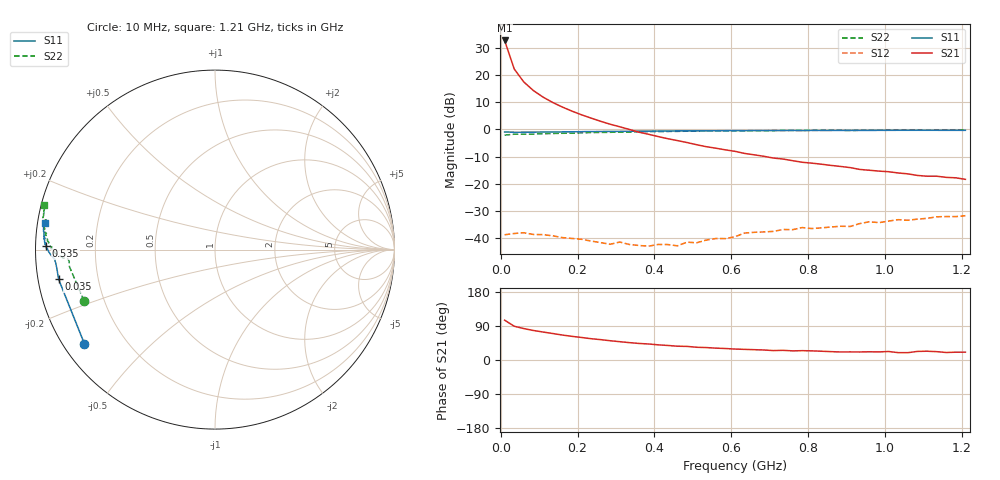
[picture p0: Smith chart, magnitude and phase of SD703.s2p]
!  POLYFET RF DEVICES
!  S PARAMETERS FOR
!  SD703 (EACH SIDE)
!  VDS=28, IDQ=600MA
! S1A3Die Vds=28Vdc, Idq=600ma, Vgsth=2.63Vdc
! Date: Thu Jul 23 11:57:09 1998
# MHZ  S  MA  R  50.0000
! SCATTERING PARAMETERS :
! Freq=MHz Mag[s11] Ang[s11] Mag[s21] Ang[s21] Mag[s12] Ang[s12] Mag[s22] Ang[s22]
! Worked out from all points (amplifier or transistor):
!   49 points, 10 MHz to 1.21 GHz, reference 50 ohm
!   highest |S21| = 32.7 dB at 10 MHz (marker M1)
!   |S21| within 3 dB of that: start of sweep to 17.16 MHz
!   unconditionally stable (mu >= 1): 240.9 MHz to 1.198 GHz
!   at 210 MHz: K = 0.81, MSG = 22.9 dB, |S12| = -40.3 dB
!   at 610 MHz: K = 1.64, MAG = 11.0 dB, |S12| = -39.4 dB
!   at 1.21 GHz: K = 0.90, MSG = 6.7 dB, |S12| = -31.7 dB
!   S11 on the Smith chart (normalised r, x): 10 MHz: 0.06, -0.32; 35 MHz: 0.06, -0.09; 535 MHz: 0.03, +0.01; 1.21 GHz: 0.02, +0.08
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10  0.897 -144.2  42.98 105.2  0.01161 14.4  0.7836 -158.6
35  0.8869 -169.3  12.86 89.1  0.01225 6.7  0.8165 -173.3
60  0.8875 -173.4  7.428 82.9  0.01266 0.6  0.8157 -175.6
85  0.8905 -175.2  5.163 77.9  0.01176 1.9  0.8214 -176.4
110  0.8936 -176.0  3.922 73.9  0.01167 -1.3  0.8317 -176.5
135  0.8939 -176.5  3.127 70.0  0.01112 2.0  0.84 -176.7
160  0.9003 -176.8  2.581 65.9  0.01032 0.3  0.8485 -176.8
185  0.9022 -177.3  2.172 62.5  0.00994 -1.5  0.853 -177.1
210  0.9078 -177.6  1.858 59.5  0.00961 -1.5  0.8621 -177.5
235  0.912 -177.8  1.613 56.2  0.0089 6.6  0.8759 -177.7
285  0.9173 -178.4  1.244 50.8  0.00777 10.7  0.8843 -178.4
310  0.9212 -178.7  1.117 48.3  0.00854 14.7  0.8942 -178.9
360  0.9271 -179.2  0.8884 43.7  0.00738 29.0  0.9018 -179.9
410  0.9312 -179.8  0.738 40.0  0.00771 35.4  0.9102 179.0
460  0.9395 179.6  0.6231 36.4  0.00727 41.4  0.9202 178.6
485  0.9388 179.2  0.5738 35.9  0.0085 52.2  0.9264 177.7
535  0.9407 178.7  0.4815 32.8  0.00928 62.5  0.935 177.0
610  0.9489 178.2  0.3957 28.8  0.0107 73.1  0.9404 175.6
635  0.9466 177.6  0.362 28.1  0.01248 74.5  0.9462 175.1
810  0.957 175.7  0.24 24.1  0.0151 79.5  0.9609 172.3
1010  0.9611 173.6  0.1671 22.5  0.0207 87.6  0.9752 169.4
1210  0.9606 171.2  0.121 20.6  0.02602 79.9  0.9848 165.5
